{attribute 'Tc2GvlVarNames'}
(*配方功能相关变量*)
VAR_GLOBAL
	g_sRecipeCtrl				: ST_RecipeCtrl_2;
END_VAR

VAR_GLOBAL CONSTANT
	MAX_RECIPE_NUM				: INT := 15;	(*配方列表中显示的文件数量*)
	MAX_RECIPE_DATA				: INT := 2;	(*配方变量(一个结构、数组只算一个变量, 离散的)*)
END_VAR
